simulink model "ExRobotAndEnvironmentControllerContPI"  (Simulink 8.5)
settings: Solver=ode45  StartTime=0.0  StopTime=1000  FixedStep=.01  RelTol=1e-3
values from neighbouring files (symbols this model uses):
  INITIAL_ROBOT_POS_THETA = 1.5*2    (= 3)    [InitRobotAndEnvironment.m]
  INITIAL_ROBOT_POS_X = 0    [InitRobotAndEnvironment.m]
  INITIAL_ROBOT_POS_Y = 0    [InitRobotAndEnvironment.m]
  INTER_WHEEL_DISTANCE = 0.12    [InitRobotAndEnvironment.m]
  ki_teta = omega*omega/alpha    (= 0.2)    [sampling.m]    (also in InitRobotAndEnvironment.m = 0.12)
  kp_teta = 2*ksi*omega/alpha    (= 0.4)    [sampling.m]    (also in InitRobotAndEnvironment.m = 0.36)
  MAX_SPEED = .5    (= 0.5)    [InitRobotAndEnvironment.m]
  ts = SENSOR_SAMPLING_TIME    (= 0.001)    [InitRobotAndEnvironment.m]
  ts_anim = ANIMATION_SAMPLING_TIME    (= 0.01)    [InitRobotAndEnvironment.m]
undefined symbols (not defined in the file or in its folder): Env, Robot, RobotInit

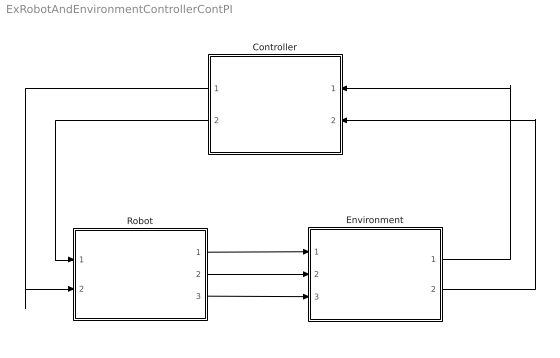
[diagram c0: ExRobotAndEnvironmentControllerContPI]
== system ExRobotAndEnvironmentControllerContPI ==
  Controller : Subsystem
  Environment : Subsystem
  Robot : Subsystem
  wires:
  Robot/1(x) -> Environment/1(x)
  Robot/2(y) -> Environment/2(y)
  Robot/3(theta) -> Environment/3(theta)
  Environment/1(Cg) -> Controller/1(Cg)
  Environment/2(Cd) -> Controller/2(Cd)
  Controller/1(v_d) -> Robot/2(v_g)
  Controller/2(v_g) -> Robot/1(v_d)

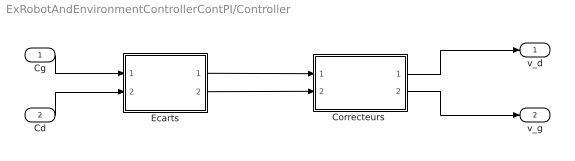
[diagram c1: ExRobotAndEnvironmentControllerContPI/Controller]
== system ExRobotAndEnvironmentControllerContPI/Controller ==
  Cg : Inport
  Cd : Inport  Port=2
  "Correcteurs " : Subsystem
  Ecarts : Subsystem
  v_d : Outport
  v_g : Outport  Port=2
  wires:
  "Correcteurs "/2(v_g) -> v_g/1
  "Correcteurs "/1(v_d) -> v_d/1
  Ecarts/2(eps_delta) -> "Correcteurs "/2(eps_delta)
  Cg/1 -> Ecarts/1(Cg)
  Cd/1 -> Ecarts/2(Cd)
  Ecarts/1(eps_teta) -> "Correcteurs "/1(eps_teta)

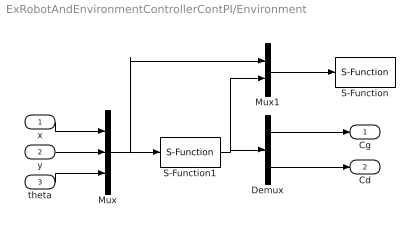
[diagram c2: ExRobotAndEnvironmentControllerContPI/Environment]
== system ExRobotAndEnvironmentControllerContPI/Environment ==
  x : Inport
  y : Inport  Port=2
  theta : Inport  Port=3
  Demux : Demux  Outputs=2
  Mux : Mux  Inputs=3
  Mux1 : Mux  Inputs=2
  S-Function : S-Function  FunctionName=robot_anim  Parameters=ts_anim,Env,Robot,RobotInit
  S-Function1 : S-Function  FunctionName=sensors  Parameters=ts,Env,Robot
  Cg : Outport
  Cd : Outport  Port=2
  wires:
  x/1 -> Mux/1
  y/1 -> Mux/2
  theta/1 -> Mux/3
  Mux/1 -> S-Function1/1, Mux1/1
  S-Function1/1 -> Mux1/2, Demux/1
  Mux1/1 -> S-Function/1
  Demux/1 -> Cg/1
  Demux/2 -> Cd/1

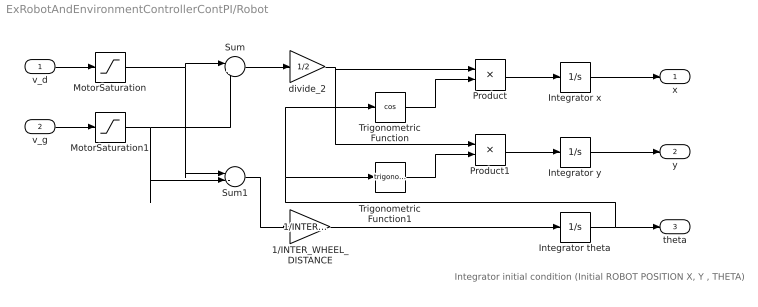
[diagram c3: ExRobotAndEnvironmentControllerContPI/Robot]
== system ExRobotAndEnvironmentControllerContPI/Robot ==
  note: Integrator initial condition (Initial ROBOT POSITION X, Y , THETA)
  v_d : Inport
  v_g : Inport  Port=2
  1/INTER_WHEEL_DISTANCE : Gain  Gain=1/INTER_WHEEL_DISTANCE
  Integrator theta : Integrator  InitialCondition=INITIAL_ROBOT_POS_THETA
  Integrator x : Integrator  InitialCondition=INITIAL_ROBOT_POS_X
  Integrator y : Integrator  InitialCondition=INITIAL_ROBOT_POS_Y
  MotorSaturation : Saturate  UpperLimit=MAX_SPEED  LowerLimit=-MAX_SPEED
  MotorSaturation1 : Saturate  UpperLimit=MAX_SPEED  LowerLimit=-MAX_SPEED
  Product : Product
  Product1 : Product
  Sum : Sum  Inputs=|++
  Sum1 : Sum  Inputs=|-+
  Trigonometric Function : Trigonometry  Operator=cos
  Trigonometric Function1 : Trigonometry
  divide_2 : Gain  Gain=1/2
  x : Outport
  y : Outport  Port=2
  theta : Outport  Port=3
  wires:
  v_d/1 -> MotorSaturation/1
  Integrator x/1 -> x/1
  Integrator y/1 -> y/1
  Integrator theta/1 -> Trigonometric Function/1, Trigonometric Function1/1, theta/1
  Sum/1 -> divide_2/1
  divide_2/1 -> Product1/1, Product/1
  Trigonometric Function/1 -> Product/2
  Trigonometric Function1/1 -> Product1/2
  Product/1 -> Integrator x/1
  Product1/1 -> Integrator y/1
  Sum1/1 -> 1/INTER_WHEEL_DISTANCE/1
  1/INTER_WHEEL_DISTANCE/1 -> Integrator theta/1
  v_g/1 -> MotorSaturation1/1
  MotorSaturation1/1 -> Sum/2, Sum1/2
  MotorSaturation/1 -> Sum/1, Sum1/1

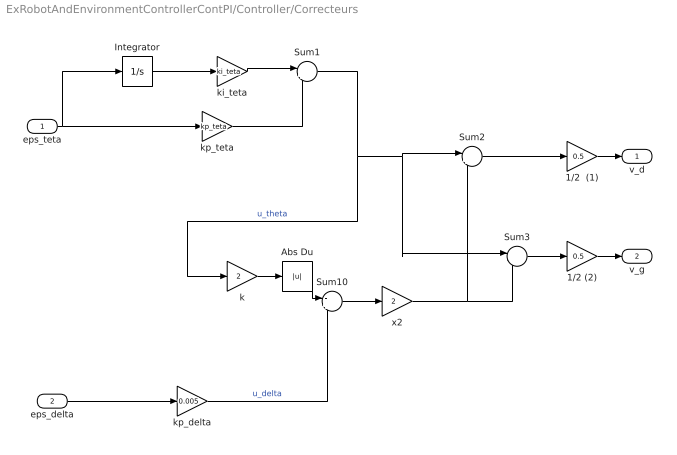
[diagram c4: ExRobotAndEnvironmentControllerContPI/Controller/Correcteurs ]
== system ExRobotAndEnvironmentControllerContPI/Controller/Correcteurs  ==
  eps_teta : Inport
  eps_delta : Inport  Port=2
  1/2  (1) : Gain  Gain=0.5
  1/2 (2) : Gain  Gain=0.5
  Abs Du : Abs
  Integrator : Integrator
  Sum1 : Sum  Inputs=|++
  Sum10 : Sum  Inputs=-+
  Sum2 : Sum  Inputs=|++
  Sum3 : Sum  Inputs=|-+
  k : Gain  Gain=2
  ki_teta : Gain  Gain=ki_teta
  kp_delta : Gain  Gain=0.005
  kp_teta : Gain  Gain=kp_teta
  x2 : Gain  Gain=2
  v_d : Outport
  v_g : Outport  Port=2
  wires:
  ki_teta/1 -> Sum1/1
  kp_teta/1 -> Sum1/2
  Sum2/1 -> 1/2  (1)/1
  Sum3/1 -> 1/2 (2)/1
  k/1 -> Abs Du/1
  kp_delta/1 -> Sum10/2  "u_delta"
  eps_teta/1 -> kp_teta/1, Integrator/1
  Abs Du/1 -> Sum10/1
  x2/1 -> Sum2/2, Sum3/2
  Sum10/1 -> x2/1
  Sum1/1 -> k/1, Sum2/1, Sum3/1  "u_theta"
  1/2  (1)/1 -> v_d/1
  1/2 (2)/1 -> v_g/1
  eps_delta/1 -> kp_delta/1
  Integrator/1 -> ki_teta/1

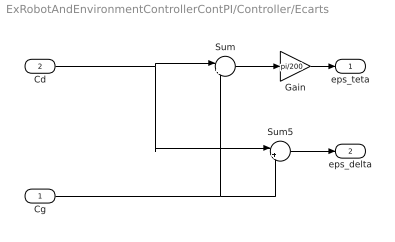
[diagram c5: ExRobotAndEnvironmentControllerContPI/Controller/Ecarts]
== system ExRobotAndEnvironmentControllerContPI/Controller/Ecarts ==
  Cg : Inport
  Cd : Inport  Port=2
  Gain : Gain  Gain=pi/200
  Sum : Sum  Inputs=|+-
  Sum5 : Sum  Inputs=|++
  eps_teta : Outport
  eps_delta : Outport  Port=2
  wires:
  Sum/1 -> Gain/1
  Cd/1 -> Sum/1, Sum5/1
  Cg/1 -> Sum/2, Sum5/2
  Gain/1 -> eps_teta/1
  Sum5/1 -> eps_delta/1
